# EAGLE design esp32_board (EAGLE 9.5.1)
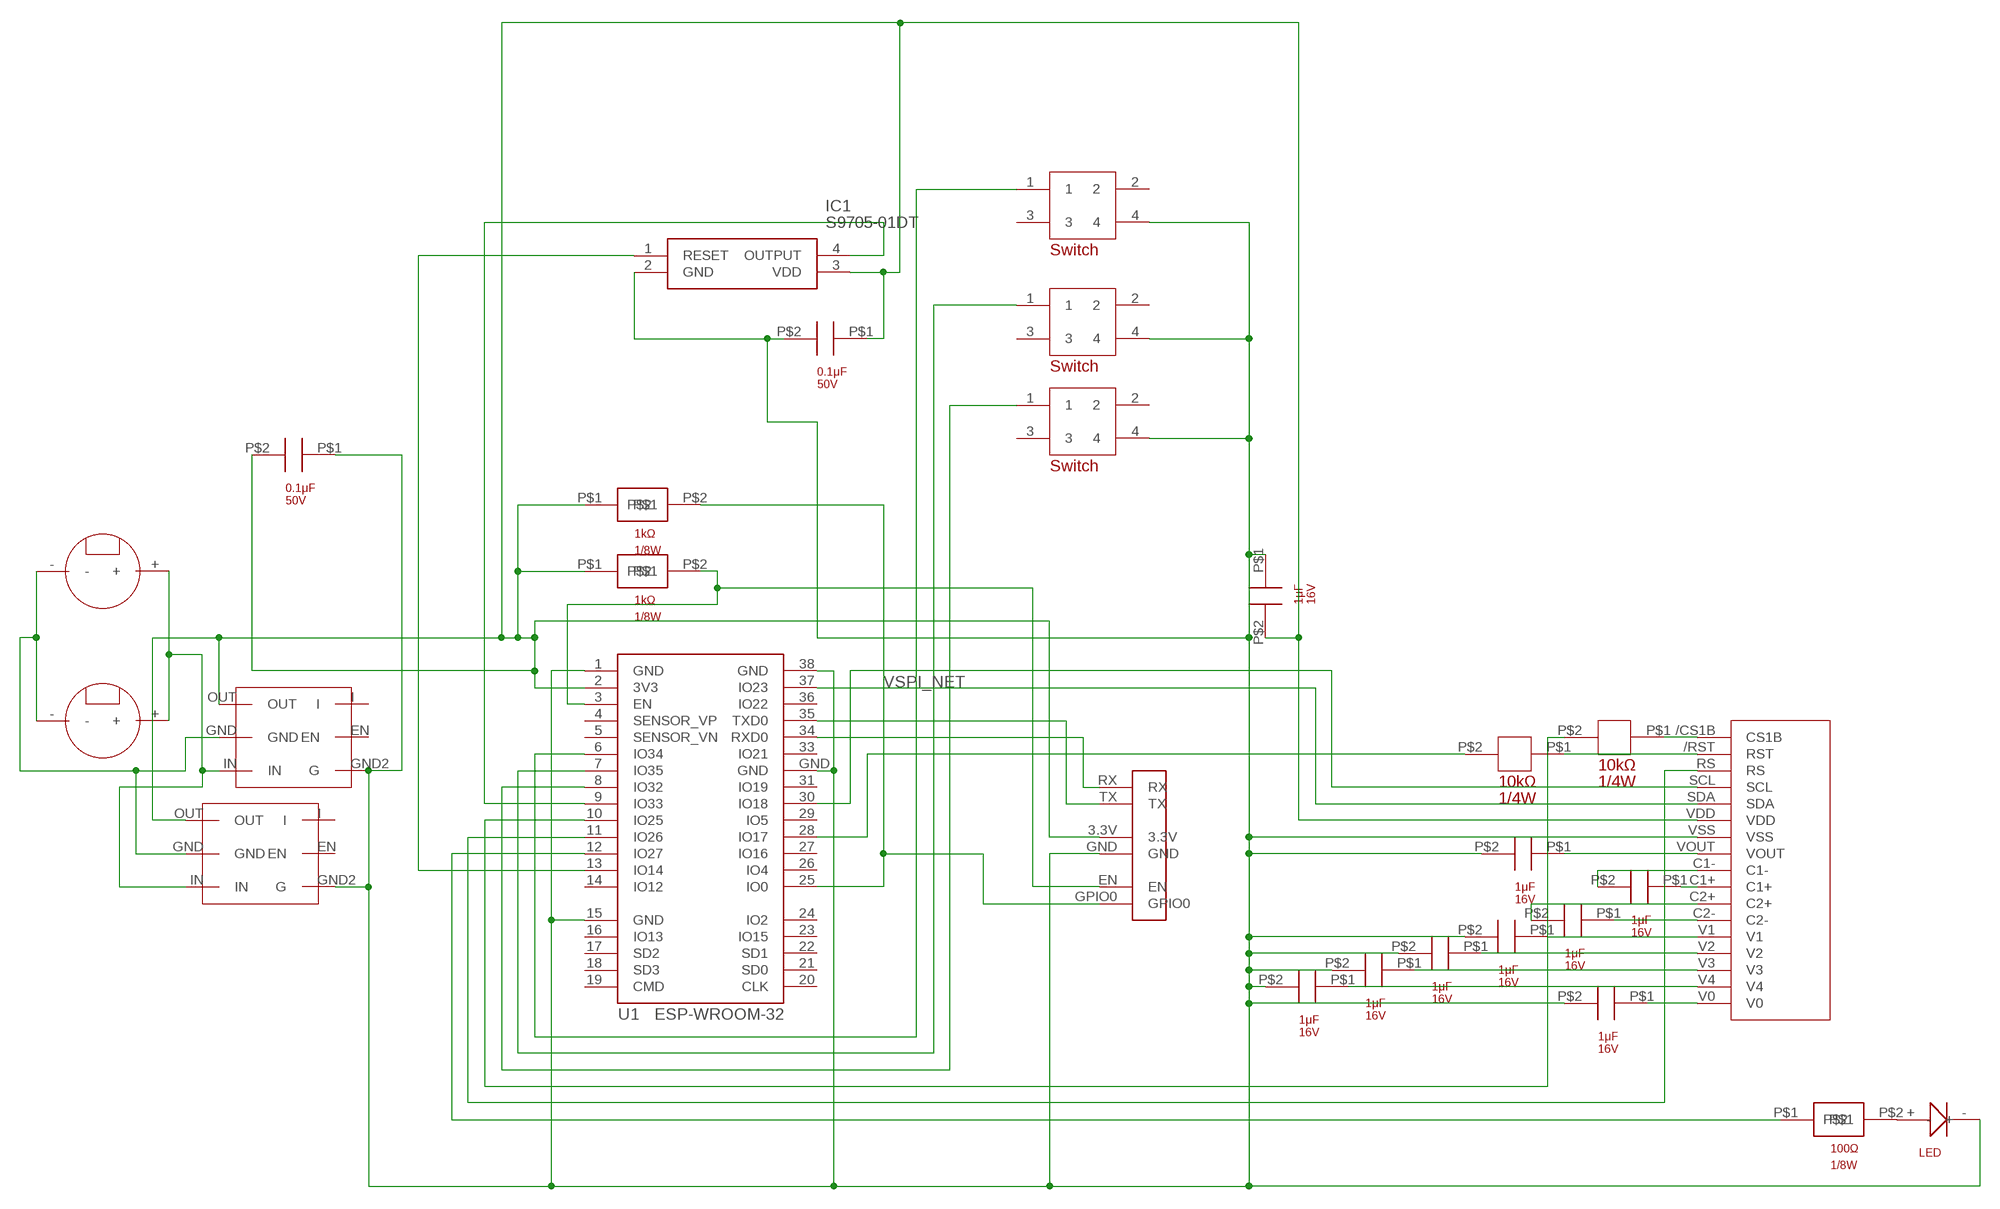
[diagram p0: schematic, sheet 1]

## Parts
AQM1  AQM1248  [AQM1248]
IC1  S9705-01DT  [SOP254P500X130-4N]
U1  ESP-WROOM-32  [ESP-WROOM-32]
U$1  3.3V_CONVERTER  [3.3V_CONVERTER]
U$2  CR2032  [CR2032]
U$3  CR2032  [CR2032]
U$4  SMD_TACT_SWITCH  [SMD_TACT_SWITCH]
U$5  SMD_TACT_SWITCH  [SMD_TACT_SWITCH]
U$6  SMD_TACT_SWITCH  [SMD_TACT_SWITCH]
U$7  1608_SC_1μF  [1608_SC_1μF]
U$8  1608_SC_1μF  [1608_SC_1μF]
U$9  1608_SC_1μF  [1608_SC_1μF]
U$10  1608_SC_1μF  [1608_SC_1μF]
U$11  1608_SC_1μF  [1608_SC_1μF]
U$12  1608_SC_1μF  [1608_SC_1μF]
U$13  1608_SC_1μF  [1608_SC_1μF]
U$14  1608_SC_1μF  [1608_SC_1μF]
U$15  1608_SC_1μF  [1608_SC_1μF]
U$16  RG3216  [RG3216]
U$17  RG3216  [RG3216]
U$18  CONNECTOR_UART  [CONNECTOR_UART]
U$19  RG2012_1KΩ  [RG2012_1KΩ]
U$20  RG2012_1KΩ  [RG2012_1KΩ]
U$21  RG2012_100Ω  [RG2012_100Ω]
U$22  LED  [LED]
U$23  1005_SC_0.1μF  [1005_SC_0.1μF]
U$24  1005_SC_0.1μF  [1005_SC_0.1μF]
U$25  3.3V_CONVERTER  [3.3V_CONVERTER]

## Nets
3.3V [pLine]: AQM1.VDD IC1.3(VDD) U1.2(3V3) U$1.OUT U$15.P$2 U$18.3.3V U$19.P$1 U$20.P$1 U$23.P$1 U$24.P$2 U$25.OUT
B_GND [pLine]: U$1.GND U$2.- U$3.- U$25.GND
B_VCC [pLine]: U$1.IN U$2.+ U$3.+ U$25.IN
N$1 [P_register]: AQM1.C1+ U$7.P$1
N$3: IC1.1(RESET) U1.13(IO14)
N$5 [P_register]: AQM1.C1- U$7.P$2
N$6 [P_register]: AQM1.C2- U$8.P$1
N$7 [P_register]: AQM1.C2+ U$8.P$2
N$8 [P_register]: AQM1.V1 U$9.P$1
N$9 [P_register]: AQM1.V2 U$10.P$1
N$10 [P_register]: AQM1.V3 U$11.P$1
N$11 [P_register]: AQM1.V4 U$12.P$1
N$12 [P_register]: AQM1.V0 U$13.P$1
N$13: AQM1.VOUT U$14.P$1
N$14: AQM1.SDA U1.37(IO23)
N$15: AQM1./CS1B(CS1B) U$16.P$1
N$16: AQM1./RST(RST) U$17.P$1
N$17: AQM1.RS U1.11(IO26)
N$18: U1.12(IO27) U$21.P$1
N$19: IC1.4(OUTPUT) U1.9(IO33)
N$20: U1.28(IO17) U$17.P$2
N$22: U1.6(IO34) U$6.1
N$23: U1.7(IO35) U$4.1
N$24: U1.8(IO32) U$5.1
N$25: U1.35(TXD0) U$18.TX
N$26: U1.34(RXD0) U$18.RX
N$27: U1.10(IO25) U$16.P$2
N$28: U1.25(IO0) U$18.GPIO0 U$20.P$2
N$29: U$21.P$2 U$22.+
N$31: U1.3(EN) U$18.EN U$19.P$2
SGND [pLine]: AQM1.VSS IC1.2(GND) U1.1(GND) U1.15(GND) U1.38(GND) U1.GND U$1.GND2(G) U$4.4 U$5.4 U$6.4 U$9.P$2 U$10.P$2 U$11.P$2 U$12.P$2 U$13.P$2 U$14.P$2 U$15.P$1 U$18.GND U$22.- U$23.P$2 U$24.P$1 U$25.GND2(G)
VSPI_NET: AQM1.SCL U1.30(IO18)
Unconnected: U1.4(SENSOR_VP) U1.5(SENSOR_VN) U1.14(IO12) U1.16(IO13) U1.17(SD2) U1.18(SD3) U1.19(CMD) U1.20(CLK) U1.21(SD0) U1.22(SD1) U1.23(IO15) U1.24(IO2) U1.26(IO4) U1.27(IO16) U1.29(IO5) U1.31(IO19) U1.33(IO21) U1.36(IO22) U$1.EN U$1.I U$4.2 U$4.3 U$5.2 U$5.3 U$6.2 U$6.3 U$25.EN U$25.I

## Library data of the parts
AQM1 = Fab lib:AQM1248
IC1 = S9705-01DT:S9705-01DT: LIGHT TO FREQUENCY CONVERTER PHOTO IC Source: Datasheet; DESCRIPTION: LIGHT TO FREQUENCY CONVERTER PHOTO IC; HEIGHT: 1.3mm; MANUFACTURER_NAME: Hamamatsu; MANUFACTURER_PART_NUMBER: S9705-01DT
U1 = esp32:ESP-WROOM-32: Espressif Systems ESP-WROOM-32
U$1 U$25 = Fab lib:3.3V_CONVERTER
U$2 U$3 = Fab lib:CR2032
U$4-U$6 = Fab lib:SMD_TACT_SWITCH
U$7-U$15 = Fab lib:1608_SC_1μF
U$16 U$17 = Fab lib:RG3216
U$18 = Fab lib:CONNECTOR_UART
U$19 U$20 = Fab lib:RG2012_1KΩ
U$21 = Fab lib:RG2012_100Ω
U$22 = Fab lib:LED
U$23 U$24 = Fab lib:1005_SC_0.1μF

## Module MOSI
Ports: 

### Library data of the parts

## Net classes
0 signal: width 0.178 mm, drill 0.4 mm, clearance 0.152 mm
1 P_register: width 0.178 mm, drill 0.4 mm, clearance 0.152 mm
2 pLine: width 0.381 mm, clearance 0.229 mm
3 ESP32: width 0.254 mm, clearance 0.203 mm

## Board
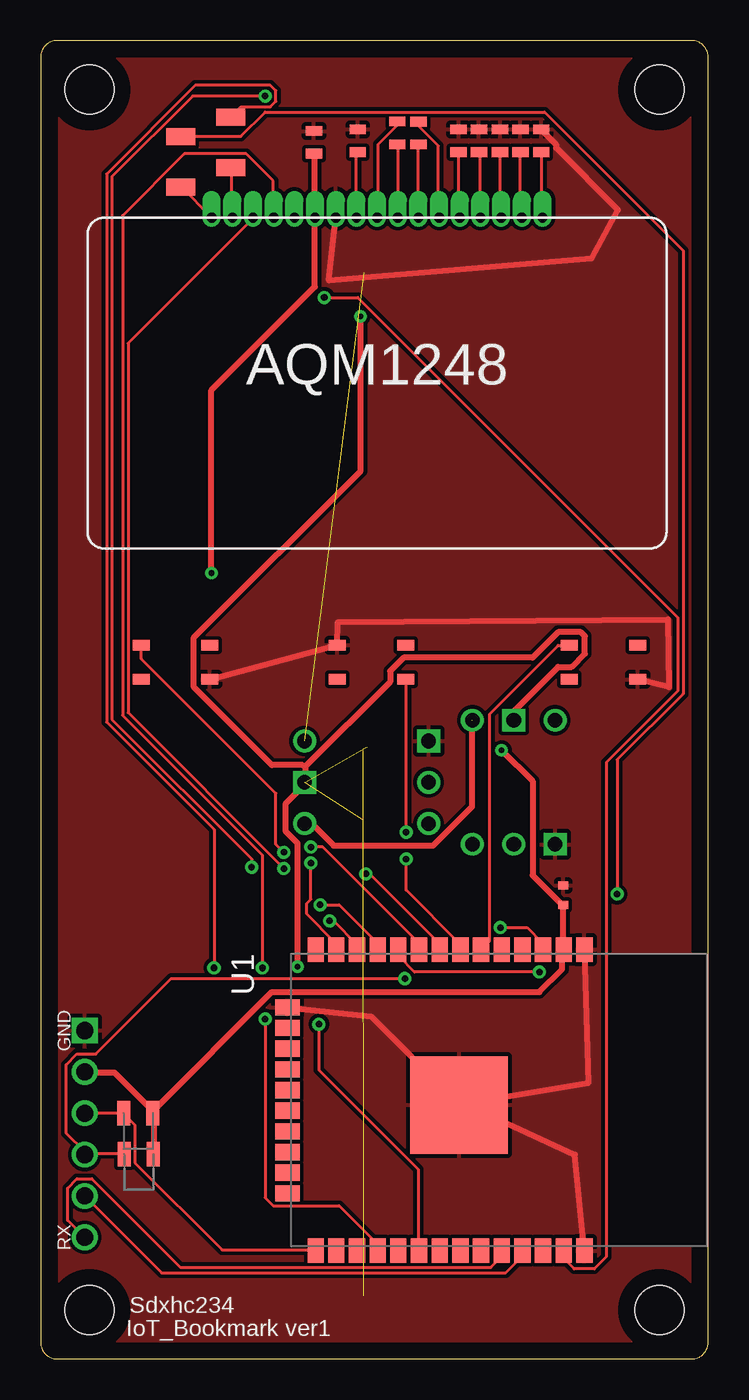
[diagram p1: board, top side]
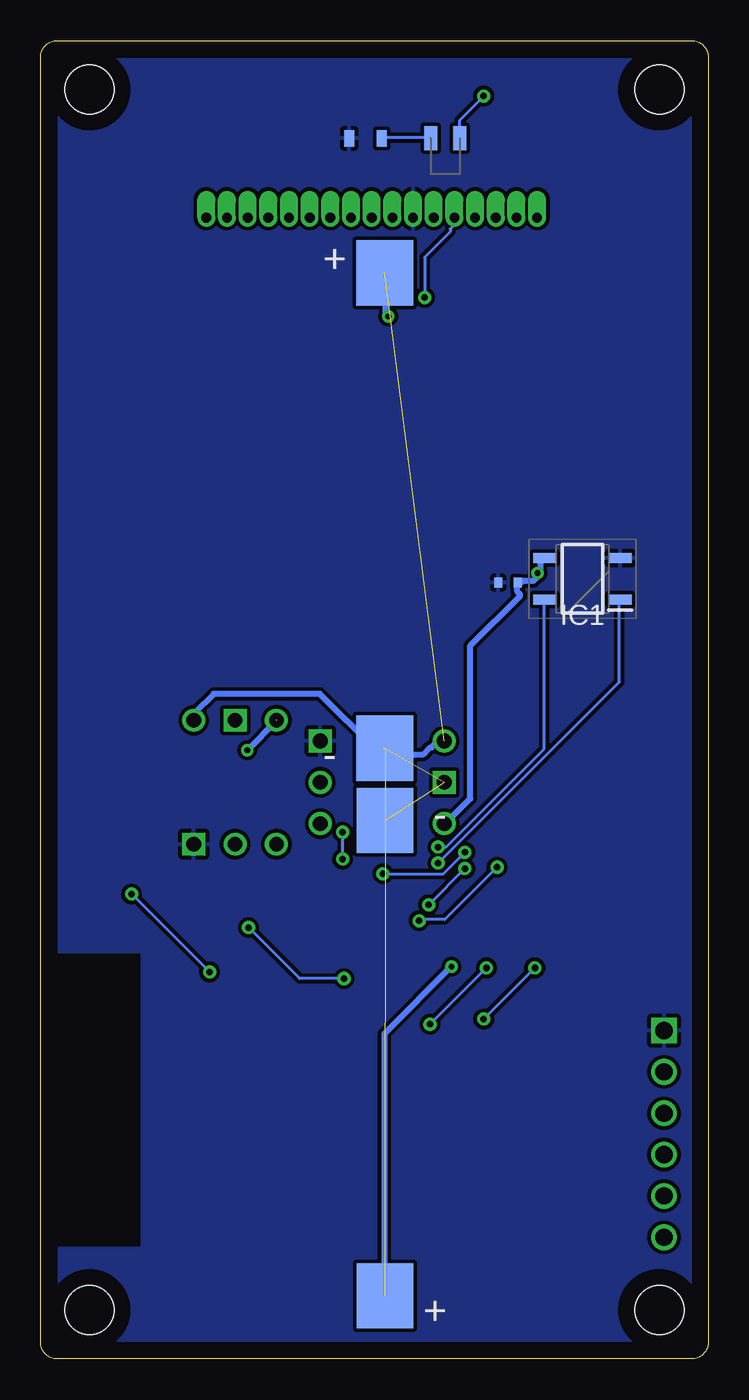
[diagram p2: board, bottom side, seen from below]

Size 41 x 81 mm. Coordinates in mm from the lower left corner, seen from the top.
Outline: 0,80 0,1 arc90 1,0 40,0 arc90 41,1 41,80 arc90 40,81 1,81 arc90 0,80
Copper layers (1*16): Top 0.035mm / dielectric 1.13mm / Bottom 0.035mm
Design rules "default *": minimum track width 6mil, minimum drill 0.35mm, track to track 6mil, track to pad 6mil, pad to pad 6mil, via to via 6mil, smd to smd 6mil, copper to edge 40mil, drill to drill 6mil, minimum pad ring 10mil, minimum via ring 8mil, stop-mask expansion 4mil, vias tented up to drill 0mil, thermal gap 10mil
Holes 3 mm at 3,78 38,78 3,3 38,3

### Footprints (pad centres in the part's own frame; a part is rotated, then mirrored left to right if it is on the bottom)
AQM1248 = drill 0.6 pad 0.33 offset: /CS1B 10.16,0; /RST 8.89,0; C1+ -1.27,0; C1- 0,0; C2+ -2.54,0; C2- -3.81,0; RS 7.62,0; SCL 6.35,0; SDA 5.08,0; V0 -10.16,0; V1 -5.08,0; V2 -6.35,0; V3 -7.62,0; V4 -8.89,0; VDD 3.81,0; VOUT 1.27,0; VSS 2.54,0
SOP254P500X130-4N = smd 1.425 x 0.6: 1 -2.312,1.27; 2 -2.312,-1.27; 3 2.312,-1.27; 4 2.312,1.27
ESP-WROOM-32 = smd 1.5 x 1: 1 -9.25,7; 2 -9.25,5.73; 3 -9.25,4.46; 4 -9.25,3.19; 5 -9.25,1.92; 6 -9.25,0.65; 7 -9.25,-0.62; 8 -9.25,-1.89; 9 -9.25,-3.16; 10 -9.25,-4.43; 11 -9.25,-5.7; 12 -9.25,-6.97; 13 -9.25,-8.24; 14 -9.25,-9.51; 25 9.25,-9.51; 26 9.25,-8.24; 27 9.25,-6.97; 28 9.25,-5.7; 29 9.25,-4.43; 30 9.25,-3.16; 31 9.25,-1.89; 32 9.25,-0.62; 33 9.25,0.65; 34 9.25,1.92; 35 9.25,3.19; 36 9.25,4.46; 37 9.25,5.73; 38 9.25,7 | smd 1 x 1.5: 15 -5.7,-11.25; 16 -4.43,-11.25; 17 -3.16,-11.25; 18 -1.89,-11.25; 19 -0.62,-11.25; 20 0.65,-11.25; 21 1.92,-11.25; 22 3.19,-11.25; 23 4.46,-11.25; 24 5.73,-11.25 | smd 6 x 6: GND 0.3,-0.7
3.3V_CONVERTER = drill 0.9: EN 0,-5.08; I 2.54,-5.08; IN -2.54,2.54; OUT 2.54,2.54 | drill 0.9 square: GND 0,2.54; GND2 -2.54,-5.08
CR2032 = smd 3.5 x 4: + 0,11.43; - 0,-17.78
SMD_TACT_SWITCH = smd 1.05 x 0.65: 1 2.1,-3.15; 2 6.3,-3.15; 3 2.1,-5.25; 4 6.3,-5.25
1608_SC_1μF = smd 0.6 x 1: P$1 1,0; P$2 -0.4,0
RG3216 = smd 1.05 x 1.8: P$1 -3.2,0; P$2 -6.3,0
CONNECTOR_UART = drill 1.05: 3.3V 10.16,0; EN 5.08,0; GPIO0 7.62,0; RX 0,0; TX 2.54,0 | drill 1.05 square: GND 12.7,0
RG2012_1KΩ = smd 0.8 x 1.5: P$1 1,-0.2; P$2 -0.8,-0.2
RG2012_100Ω = smd 0.8 x 1.5: P$1 1,-0.2; P$2 -0.8,-0.2
LED = smd 0.6 x 1: + 1,0; - -1,0
1005_SC_0.1μF = smd 0.5 x 0.6: P$1 1.1,0; P$2 -0.1,0

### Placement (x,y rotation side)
AQM1  20.67,70.12 180 top
IC1  7.72,47.93 180 bottom
U1  26.4,15.9 270 top
U$1  18.75,35.43 270 bottom
U$2  19.87,55.3 0 bottom
U$3  19.85,15.3 180 bottom
U$4  24.52,38.6 180 top
U$5  4.08,47 0 top
U$6  30.38,47 0 top
U$7  21.9,75.63 270 top
U$8  23.2,75.02 90 top
U$9  25.67,75.15 270 top
U$10  26.92,75.15 270 top
U$11  28.22,75.15 270 top
U$12  29.47,75.15 270 top
U$13  30.74,75.15 270 top
U$14  19.47,75.15 270 top
U$15  16.78,74.45 90 top
U$16  8.6,68.8 270 top
U$17  11.68,70 270 top
U$18  2.71,7.47 90 top
U$19  5.92,12.77 0 top
U$20  5.9,15.29 0 top
U$21  16.25,75.21 0 bottom
U$22  21.05,75 0 bottom
U$23  32.1,29 270 top
U$24  11.8,47.7 180 bottom
U$25  29.06,36.7 0 bottom

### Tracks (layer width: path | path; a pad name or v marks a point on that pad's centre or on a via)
3.3V  (via drill 0.35)  (2 unrouted)
  Top 0.381: U$19.P$1 6.93,12.63 6.93,15.02 U$20.P$1 | U$20.P$1 6.93,15.27 14.2,22.54 30.63,22.54 32.03,23.94 32.03,25.01 U1.2 32.11,25.18 32.11,27.82 U$23.P$1 31.95,27.98 30.21,29.72 30.21,35.5 v28.32,37.4 | U$18.3.3V 2.72,17.58 4.54,17.58 6.77,15.35 U$20.P$1 | U$15.P$2 16.84,74.05 16.84,70.17 AQM1.VDD 16.84,69.92 16.84,65.88 10.48,59.52 v10.48,48.29 | 26.5,39.21 26.5,33.93 24.11,31.53 18,31.53 16.68,32.85 16.26,32.85 U$1.OUT
  Bottom 0.381: 10.36,48.17 10.32,48.21 10.32,49.03 10.07,49.28 IC1.3 | 10.36,48.17 10.73,47.8 11.39,47.8 11.47,47.71 11.64,47.71 U$24.P$2 11.72,47.55 11.72,47.14 11.56,46.97 11.56,46.89 14.61,43.83 14.61,34.42 16.18,32.85 U$1.OUT | v10.48,48.29 10.36,48.17 | 26.5,39.21 v28.32,37.4
B_GND  (via drill 0.35)  (2 unrouted)
  Top 0.381: 16.26,36.41 16.26,35.5 U$1.GND 16.18,35.25 15.02,34.09 15.02,32.44 15.77,31.7 v15.77,24.11 | 16.26,36.41 21.46,41.6 21.46,42.27 22.29,43.09 30.21,43.09 31.78,44.66 33.19,44.66 33.43,44.41 33.43,43.34 32.61,42.51 31.78,42.51 29.06,39.79 U$25.GND | v19.65,64.06 19.65,54.57 9.41,44.33 9.41,41.27 14.2,36.49 16.1,36.49 16.26,36.41
  Bottom 0.381: 19.89,3.88 19.89,19.98 v15.77,24.11 | 19.81,66.7 19.81,64.22 v19.65,64.06
B_VCC  (3 unrouted)
  Bottom 0.381: 19.81,37.48 19.48,37.15 17.5,37.15 17.09,37.56 17,37.56 16.68,37.89 16.26,37.89 U$1.IN | 20.06,37.56 20.55,37.56 23.86,40.86 30.38,40.86 31.53,39.71 31.53,39.29 U$25.IN
N$1
  Top 0.178: U$7.P$1 21.96,74.62 21.96,70.17 AQM1.C1+
N$3  (via drill 0.4)
  Top 0.178: v16.59,30.46 16.59,28.23 16.34,27.98 16.34,27.32 18.08,25.59 18.08,25.18 U1.13
  Bottom 0.178: v16.59,30.46 5.45,41.6 5.45,46.64 IC1.1
N$5
  Top 0.178: U$7.P$2 21.88,76.03 21.88,75.78 20.72,74.62 20.72,70.17 AQM1.C1-
N$6
  Top 0.178: U$8.P$1 23.28,75.95 23.28,75.7 24.43,74.54 24.43,70.17 AQM1.C2-
N$7
  Top 0.178: U$8.P$2 23.2,74.54 23.2,70.17 AQM1.C2+
N$8
  Top 0.178: U$9.P$1 25.67,74.13 25.67,70.17 AQM1.V1
N$9
  Top 0.178: U$10.P$1 26.99,74.13 26.99,70.17 AQM1.V2
N$10
  Top 0.178: U$11.P$1 28.23,74.13 28.23,70.17 AQM1.V3
N$11
  Top 0.178: U$12.P$1 29.47,74.13 29.47,70.25 29.55,70.17 AQM1.V4
N$12
  Top 0.178: U$13.P$1 30.79,74.13 30.79,70.17 AQM1.V0
N$13
  Top 0.178: U$14.P$1 19.4,74.13 19.4,70.17 AQM1.VOUT
N$14  (via drill 0.4)
  Top 0.178: v17.42,65.22 19.48,65.22 39.13,45.57 39.13,41.03 34.75,36.65 34.75,6.27 34.01,5.53 32.77,5.53 32.19,6.11 32.19,6.6 U1.37
  Bottom 0.178: v17.42,65.22 17.42,67.69 15.85,69.26 15.85,69.42 15.6,69.67 15.6,70.08 AQM1.SDA
N$15
  Top 0.178: U$16.P$1 8.67,71.98 10.48,70.17 AQM1./CS1B
N$16
  Top 0.178: U$17.P$1 11.72,73.14 11.72,70.17 AQM1./RST
N$17  (via drill 0.4)
  Top 0.178: v17.17,27.9 18.33,27.9 20.64,25.59 20.64,25.18 U1.11 | v14.94,30.13 5.37,39.71 5.37,62.41 13.04,70.08 AQM1.RS
  Bottom 0.178: v14.94,30.13 v17.17,27.9
N$18  (via drill 0.4)
  Top 0.178: v17.75,26.91 18,26.91 19.4,25.51 19.4,25.18 U1.12 | v12.96,30.21 12.96,30.71 4.38,39.29 4.38,72.64 9.33,77.6 v13.79,77.6
  Bottom 0.178: v17.75,26.91 17.67,26.99 16.18,26.99 v12.96,30.21 | v13.79,77.6 15.27,76.11 15.27,75.04 U$21.P$1
N$19  (via drill 0.4)
  Top 0.178: v16.59,31.45 17.34,31.45 23.2,25.59 23.2,25.18 U1.9
  Bottom 0.178: v16.59,31.45 16.1,31.45 10.07,37.48 10.07,46.64 IC1.4
N$20  (via drill 0.4)
  Top 0.178: v13.79,20.89 13.79,9.91 14.28,9.41 18.33,9.41 20.64,7.1 20.64,6.69 U1.28 | v10.65,24.02 10.65,32.52 4.04,39.13 4.04,72.81 9.49,78.26 14.12,78.26 14.45,77.93 14.45,77.27 14.12,76.94 12.3,76.94 11.72,76.36 U$17.P$2
  Bottom 0.178: v10.65,24.02 v13.79,20.89
N$22
  Top 0.178: U$6.1 32.44,43.83 31.78,43.83 27.57,39.62 27.57,25.67 27.08,25.18 U1.6
N$23  (via drill 0.4)
  Top 0.178: v22.45,32.36 22.45,41.69 U$4.1 | v22.45,30.71 22.45,28.81 25.76,25.51 25.76,25.18 U1.7
  Bottom 0.178: v22.45,30.71 v22.45,32.36
N$24  (via drill 0.4)
  Top 0.178: v14.94,31.12 14.45,31.62 14.45,34.75 6.19,43.01 6.19,43.83 U$5.1 | v19.98,29.8 20.23,29.8 24.43,25.59 24.43,25.18 U1.8
  Bottom 0.178: v14.94,31.12 16.26,29.8 v19.98,29.8
N$25
  Top 0.178: U1.35 29.55,6.6 29.55,6.27 28.56,5.28 7.43,5.28 2.72,9.99 U$18.TX
N$26
  Top 0.178: U1.34 28.32,6.6 28.32,6.27 27.65,5.61 8.59,5.61 3.14,11.06 2.23,11.06 1.65,10.48 1.65,8.5 2.64,7.51 U$18.RX
N$27  (via drill 0.4)
  Top 0.178: v30.63,23.77 22.95,23.77 22.04,24.68 22.04,25.09 U1.10 | v35.41,28.56 35.41,36.82 39.46,40.86 39.46,68.1 30.96,76.61 13.79,76.61 12.3,75.12 8.67,75.12 U$16.P$2
  Bottom 0.178: v35.41,28.56 v30.63,23.77
N$28
  Top 0.178: U$18.GPIO0 2.72,15.11 5.04,15.11 U$20.P$2 5.12,15.02 5.78,14.36 5.78,12.05 11.14,6.69 16.84,6.69 U1.25
N$29
  Bottom 0.178: U$22.+ 19.98,75.04 17.09,75.04 U$21.P$2
N$31  (via drill 0.4)
  Top 0.178: U$19.P$2 5.12,12.63 2.72,12.63 U$18.EN 2.72,12.71 1.57,13.87 1.57,18.08 2.23,18.74 3.38,18.74 8.01,23.36 v22.37,23.36 | v28.23,26.5 29.88,26.5 30.79,25.59 30.79,25.18 U1.3
  Bottom 0.178: v28.23,26.5 25.09,23.36 v22.37,23.36
SGND
  Top 0.381: U$5.4 U$4.4 18.26,45.26 38.53,45.44 38.58,41.27 U$6.4 | U1.1 33.63,16.94 U1.GND 25.3,16 | U1.15 20.3,21.03 25.3,16 | U1.38 32.82,12.55 25.3,16 | U$13.P$2 31.66,74.62 31.66,74.41 35.46,70.61 33.83,67.61 17.7,66.27 AQM1.VSS
  pour Bottom: 39.9,79.9 39.9,1.1 0.5,1.1 0.5,79.9
  pour Top: 0.8,80 40.5,80 40.5,0.2 0.8,0.2
VSPI_NET  (via drill 0.4)
  Top 0.178: v17.09,20.55 17.09,17.75 23.2,11.64 23.2,6.69 U1.30 | v13.62,24.02 13.62,30.96 5.04,39.54 5.04,70.25 8.83,74.05 12.63,74.05 14.28,72.4 14.28,70.17 AQM1.SCL
  Bottom 0.178: v13.62,24.02 v17.09,20.55

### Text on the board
tPlace: Sdxhc234 | IoT_Bookmark ver1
